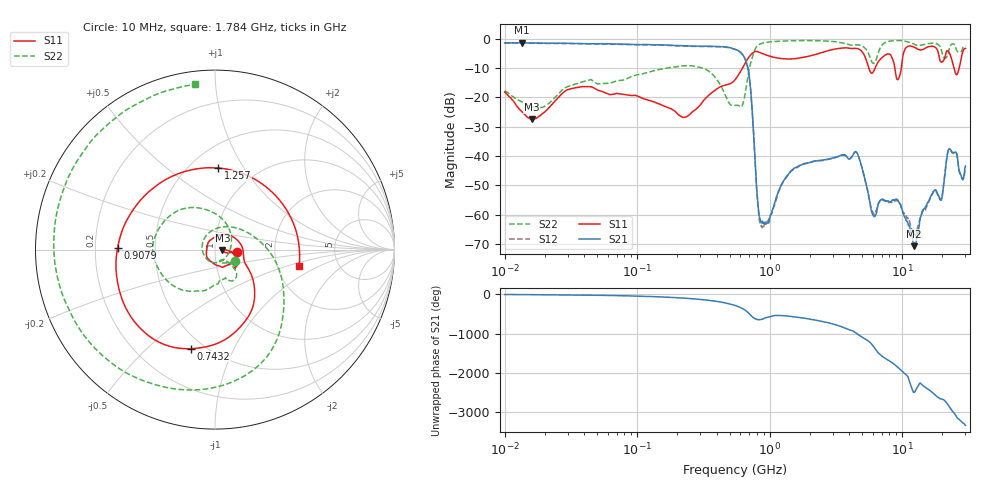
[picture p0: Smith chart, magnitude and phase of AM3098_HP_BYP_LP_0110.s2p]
!Agilent Technologies,E8364B,MY43040894,A.07.50.67
!Agilent E8364B: A.07.50.67
!Date: Wednesday, June 17, 2020 09:20:33
!Correction: S11(Full 2 Port(1,2))
!S21(Full 2 Port(1,2))
!S12(Full 2 Port(1,2))
!S22(Full 2 Port(1,2))
!S2P File: Measurements: S11, S21, S12, S22:Log Frequency Sweep
# Hz S  dB  R 50
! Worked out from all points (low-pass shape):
!   1601 points, 10 MHz to 30 GHz, reference 50 ohm
!   highest |S21| = -1.40 dB at 13.57 MHz (marker M1); lowest = -70.8 dB at 12.25 GHz (marker M2)
!   |S21| within 3 dB of the highest: start of sweep to 594.3 MHz
!   lowest |S11| = -27.6 dB at 16.01 MHz (marker M3), VSWR 1.09, Z = 54.3 - j0.457 ohm
!   |S11| at or under -10 dB: 5.592 GHz to 6.256 GHz (663.7 MHz wide, 11.2 % of centre); 8.799 GHz to 9.856 GHz (1.057 GHz wide, 11.3 % of centre); 24.61 GHz to 26.94 GHz (2.33 GHz wide, 9.04 % of centre)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
!   |S22| runs from -23.6 to -0.6 dB; largest |S21 - S12| = 0.02
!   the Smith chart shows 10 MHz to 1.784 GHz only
!   S11 on the Smith chart (normalised r, x): 10 MHz: 1.28, -0.03; 743.2 MHz: 0.43, -0.69; 907.9 MHz: 0.30, +0.01; 1.257 GHz: 0.68, +0.78; 1.784 GHz: 2.65, -0.63
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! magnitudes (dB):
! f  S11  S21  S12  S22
! 10 MHz  -18.2  -1.5  -1.5  -17.8
! 13.57 MHz  -25.0  -1.4  -1.5  -21.7
! 16.01 MHz  -27.6  -1.5  -1.5  -23.1
! 38.04 MHz  -16.4  -1.7  -1.7  -14.8
! 144.7 MHz  -22.2  -2.1  -2.2  -10.6
! 327.1 MHz  -20.4  -2.6  -2.7  -10.4
! 547.7 MHz  -14.1  -3.6  -3.7  -22.7
! 672.5 MHz  -7.3  -8.5  -8.6  -15.2
! 743.2 MHz  -4.9  -26.4  -26.5  -6.1
! 825.6 MHz  -4.6  -58.7  -60.0  -2.1
! 907.9 MHz  -5.3  -62.7  -63.7  -1.4
! 1.257 GHz  -6.8  -48.9  -49.0  -0.8
! 1.784 GHz  -6.4  -42.7  -42.9  -0.7
! 2.084 GHz  -5.7  -42.1  -42.0  -0.7
! 4.48 GHz  -3.3  -38.6  -38.6  -2.1
! 6.049 GHz  -11.4  -60.3  -59.6  -8.4
! 7.926 GHz  -5.2  -55.6  -55.9  -0.9
! 9.302 GHz  -13.9  -55.1  -55.6  -0.7
! 12.25 GHz  -2.9  -70.8  -66.9  -1.8
! 19.7 GHz  -8.0  -55.1  -54.6  -3.7
! 22.67 GHz  -4.8  -37.6  -37.9  -3.3
! 30 GHz  -3.3  -43.4  -43.9  -2.6
